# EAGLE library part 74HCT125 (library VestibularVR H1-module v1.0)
Quad buffer/line driver; 3-state
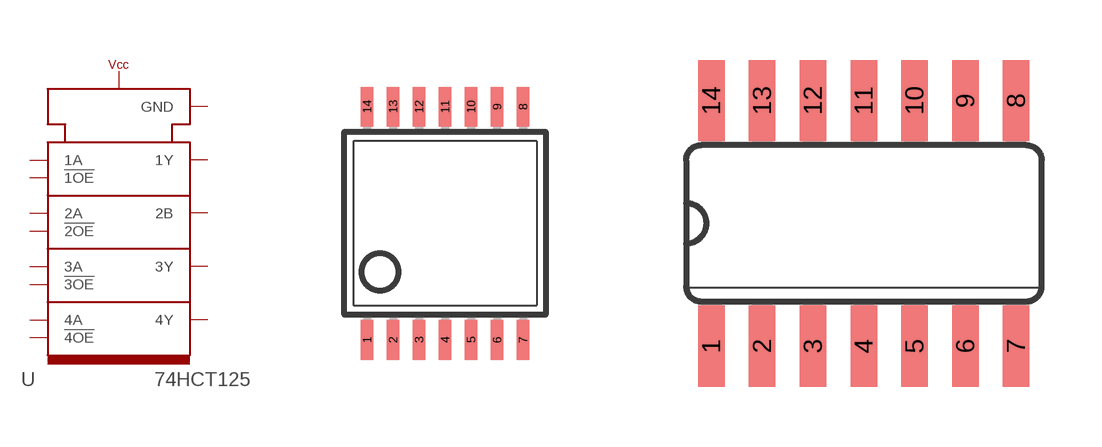
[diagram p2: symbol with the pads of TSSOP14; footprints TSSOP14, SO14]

Designator prefix U

## 74HCT125TSSOP14  [TSSOP14]
1  !1OE
2  1A
3  1Y
4  !2OE
5  2A
6  2B
7  GND
8  3Y
9  3A
10  !3OE
11  4Y
12  4A
13  !4OE
14  VCC  in

## 74HCT125SO14  [SO14]
Pads as for TSSOP14

## 74HCT125SSOP14  [SSOP14]
Pads as for TSSOP14

## Footprint TSSOP14 (pad centres in mm)
Thin Shrink Small Outline Plastic 14 MAX3223-MAX3243.pdf
smd 0.305 x 0.991: 1 -1.95,-2.918; 2 -1.3,-2.918; 3 -0.65,-2.918; 4 0,-2.918; 5 0.65,-2.918; 6 1.3,-2.918; 7 1.95,-2.918; 8 1.95,2.918; 9 1.3,2.918; 10 0.65,2.918; 11 0,2.918; 12 -0.65,2.918; 13 -1.3,2.918; 14 -1.95,2.918

## Footprint SO14 (pad centres in mm)
Small Outline package 150 mil
smd 0.66 x 2.032: 1 -3.81,-3.073; 2 -2.54,-3.073; 3 -1.27,-3.073; 4 0,-3.073; 5 1.27,-3.073; 6 2.54,-3.073; 7 3.81,-3.073; 8 3.81,3.073; 9 2.54,3.073; 10 1.27,3.073; 11 0,3.073; 12 -1.27,3.073; 13 -2.54,3.073; 14 -3.81,3.073

## Footprint SSOP14 (pad centres in mm)
plastic shrink small outline package; 14 leads; body width 5.3 mm SOT337-1 Source: http://www.nxp.com/documents/data_sheet/74ABT125.pdf
smd 0.4 x 1.1: 1 -1.95,-3.475; 2 -1.3,-3.475; 3 -0.65,-3.475; 4 0,-3.475; 5 0.65,-3.475; 6 1.3,-3.475; 7 1.95,-3.475; 8 1.95,3.475; 9 1.3,3.475; 10 0.65,3.475; 11 0,3.475; 12 -0.65,3.475; 13 -1.3,3.475; 14 -1.95,3.475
